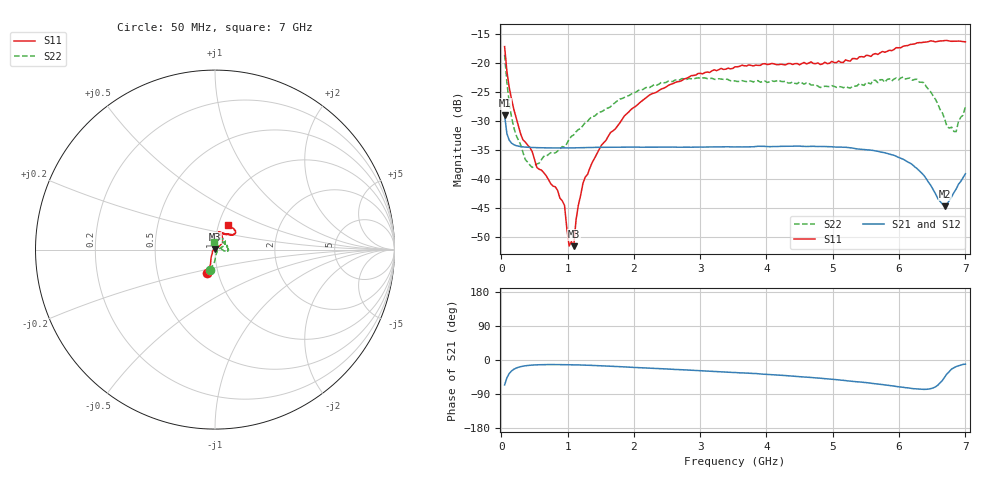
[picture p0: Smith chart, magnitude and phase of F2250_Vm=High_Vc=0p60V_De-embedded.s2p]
! Integrated Device Technology
! Corporate Headquarters
! 6024 Silver Creek Valley Road
! San Jose, CA 95138  USA
! Phone:  1-408-284-8200
! Toll Free:  1-800-223-1366
! Webpage:  http://www.idt.com/
! Timing and RF Division
! 515 Groton Road, Suite 102
! Westford, MA 01886-6024
! Device:  F2250
! Description: Voltage Variable RF Attenuator
! Frequency:  50.0 -  6000.00 MHz
! Package:  3x3 mm Thin QFN Plastic Package: 16 pin
! Ports:  2 RF, 3 DC
!  Pin  1  = GND
!  Pin  2  = NC
!  Pin  3  = RF1  = Port 1
!  Pin  4  = NC
!  Pin  5  = GND
!  Pin  6  = GND
!  Pin  7  = GND
!  Pin  8  = GND
!  Pin  9  = NC
!  Pin 10  = RF2  = Port 2
!  Pin 11  = NC
!  Pin 12  = GND
!  Pin 13  = GND
!  Pin 14  = VCNTRL
!  Pin 15  = VDD
!  Pin 16  = VMODE
! Vcntrl:  0.600 Volts
! Vmode:  +3.300 Volts
! Vdd:  +3.30  Volts
! Current:  1.277 mA
! Data:  The device was measured on a the F2250 evaluation board which has
!  individual transmission lines to the RF pins.  Data was collected
!  using a calibrated network analyzer.  The evaluation board was
!  de-embedded using a TRL calibration technique.
!  The reference plane is the edge of the package pin.
! Misc:  SN 10
!  Action Tracker AT0258
! Date Measured:  2014-11-26
! Date:  2015-10-15  MJV
! Note:
!  Integrated Device Technology supplies this data as a sample of measured
!  data at the package pin for this product.  Your particular data for this
!  product may vary.
!  Data was taken at 25 degrees C.
!  Integrated Device Technology reserves the right to change this data at anytime.
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# GHz S dB R 50
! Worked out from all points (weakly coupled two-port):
!   201 points, 50 MHz to 7 GHz, reference 50 ohm
!   highest |S21| = -29.02 dB at 50 MHz (marker M1); lowest = -44.7 dB at 6.687 GHz (marker M2)
!   lowest |S11| = -51.6 dB at 1.093 GHz (marker M3), VSWR 1.01, Z = 50 + j0.261 ohm
!   |S11| at or under -10 dB: start of sweep to end of sweep
!   |S22| runs from -38.0 to -18.6 dB; largest |S21 - S12| = 6e-05
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0.05  -17.17 -108.4  -29.02 -65.7  -29.02 -65.7  -18.60 -103.6
0.08475  -21.46 -107.2  -32.20 -46.8  -32.20 -46.8  -23.38 -91.8
0.1195  -24.21 -111.7  -33.33 -35.8  -33.34 -35.7  -26.85 -87.3
0.189  -28.01 -119.6  -34.10 -24.5  -34.10 -24.5  -31.14 -77.4
0.328  -33.29 -133.5  -34.48 -16.2  -34.49 -16.2  -35.49 -46.4
0.43225  -34.61 -144.8  -34.57 -13.9  -34.57 -13.9  -37.65 -21.8
0.5365  -38.04 -154.1  -34.62 -12.8  -34.62 -12.8  -37.43 -12.8
0.9535  -44.58 170.9  -34.67 -12.3  -34.68 -12.3  -34.55 11.4
1.023  -51.59 138.6  -34.66 -12.5  -34.66 -12.5  -33.14 12.8
1.0925  -51.62 85.2  -34.65 -12.7  -34.65 -12.7  -32.41 14.7
1.12725  -47.10 58.5  -34.63 -12.8  -34.64 -12.9  -31.86 13.1
1.2315  -40.78 39.2  -34.61 -13.3  -34.61 -13.3  -30.79 12.2
1.6485  -32.00 40.6  -34.55 -16.4  -34.55 -16.4  -27.54 21.2
2.37825  -24.75 46.4  -34.53 -22.7  -34.53 -22.7  -23.65 30.4
3.525  -20.66 71.6  -34.50 -33.0  -34.50 -33.0  -23.09 58.1
4.7065  -20.07 71.9  -34.39 -46.7  -34.39 -46.7  -23.81 60.9
5.2625  -19.68 53.1  -34.63 -55.8  -34.63 -55.9  -24.34 38.3
5.85325  -17.80 40.5  -35.73 -67.2  -35.72 -67.4  -22.72 9.4
6.3745  -16.41 40.9  -39.41 -77.5  -39.42 -77.6  -23.39 -7.2
6.68725  -16.12 47.8  -44.71 -45.1  -44.69 -44.9  -29.62 13.7
6.861  -16.23 54.4  -41.76 -17.4  -41.72 -17.5  -31.84 60.3
7  -16.34 62.4  -39.12 -11.0  -39.08 -11.2  -27.52 96.5
